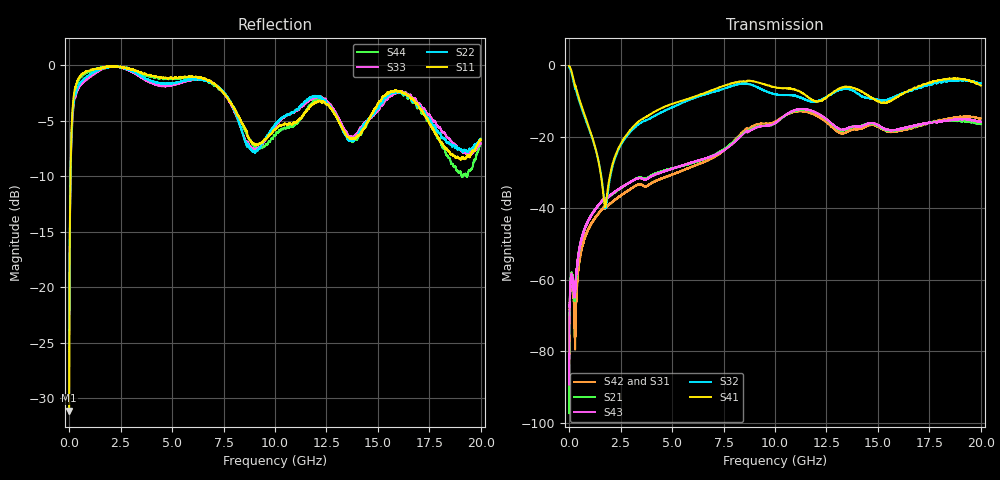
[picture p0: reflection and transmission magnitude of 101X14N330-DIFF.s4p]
!{101X14N330}
!Johanson Technology Inc.
!www.johansontechnology.com
!Test Board Conditions:
!Substrate Type  RO4350B
!Substrate Thickness  10 mil
!Substrate Dk  3.66
!TL Type: GCPW
!TL Trace Width  20 mil
!TL Gap  15 mil
!PART MODE DIFFERENTIAL
!DUT TOPOLOGY	DIFFERENTIAL 4-PORT
!Mounting Pad LxW  20x35 mil
# MHz S  dB  R 50
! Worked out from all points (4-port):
!   20001 points, 300 kHz to 20 GHz, reference 50 ohm
!   strongest paths, dB at 300 kHz, 5 GHz, 10 GHz, 15 GHz, 20 GHz:
!     S41: -0.3, -10.8, -6.1, -10.1, -5.7
!     S32: -0.6, -11.8, -8.1, -9.7, -5.0
!     S43: -83.5, -29.0, -16.2, -16.8, -15.8
!     S21: -84.0, -28.9, -16.3, -16.9, -16.5
!     S42: -77.8, -30.6, -15.8, -17.3, -14.9
!     S31: -88.9, -30.5, -15.8, -17.3, -14.9
!   lowest |S11| = -31.1 dB at 300 kHz (marker M1), VSWR 1.06, Z = 52.8 - j0.523 ohm
!   |S11| at or under -10 dB: start of sweep to 66.42 MHz
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0.3  -31.15 -10.3  -81.95 64.8  -76.57 -137.4  -0.28 0.2
     -84.03 132.1  -23.86 -3.9  -0.61 0.0  -78.14 -172.1
     -88.94 139.1  -0.63 0.2  -23.75 -4.6  -79.90 -33.1
     -0.25 0.2  -77.76 172.7  -83.54 165.1  -31.38 -9.1
262.296  -2.30 -146.2  -63.35 56.3  -70.68 24.4  -5.13 -55.8
         -64.60 54.2  -2.76 -146.5  -5.77 -56.5  -71.04 19.0
         -69.89 24.7  -5.78 -56.5  -3.02 -146.2  -63.78 67.1
         -5.15 -55.8  -68.61 11.8  -64.29 68.1  -2.39 -146.5
723.289  -0.71 -171.6  -46.25 99.8  -48.83 105.4  -13.36 -78.9
         -46.21 100.4  -1.22 -174.0  -14.01 -78.8  -48.88 105.6
         -48.93 106.9  -13.98 -78.9  -1.47 -174.5  -46.34 99.5
         -13.40 -79.0  -48.94 103.5  -46.35 99.1  -0.83 -173.9
1773.273  -0.15 170.1  -37.55 77.2  -39.80 76.3  -39.09 7.4
          -37.60 76.8  -0.23 170.5  -39.92 -3.0  -39.86 76.2
          -39.84 76.2  -39.85 -3.1  -0.24 169.8  -37.50 77.5
          -39.15 7.9  -39.80 76.8  -37.59 77.8  -0.16 170.2
3273.251  -0.50 160.7  -31.62 53.7  -33.65 47.4  -16.22 61.8
          -31.67 53.7  -0.72 160.3  -17.01 59.0  -33.56 47.9
          -33.59 47.3  -16.98 59.2  -0.83 160.2  -31.74 53.0
          -16.24 61.7  -33.56 48.0  -31.73 53.0  -0.54 160.8
7812.183  -3.27 119.7  -22.19 -34.3  -22.16 -43.5  -5.16 12.7
          -22.21 -34.4  -3.24 114.2  -6.01 6.7  -22.29 -47.6
          -22.12 -43.7  -5.95 6.5  -3.39 113.8  -22.48 -38.9
          -5.17 12.8  -22.29 -47.5  -22.57 -38.6  -3.20 113.1
20000  -6.70 79.3  -16.46 171.0  -14.91 169.8  -5.67 -82.6
       -16.46 170.9  -6.62 67.2  -5.07 -74.7  -14.85 171.9
       -14.88 170.4  -5.05 -73.9  -7.04 61.0  -15.72 170.4
       -5.69 -82.3  -14.87 172.4  -15.80 170.1  -6.99 81.2
